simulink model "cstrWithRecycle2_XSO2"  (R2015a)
settings: Solver=ode45  StartTime=0.0  StopTime=tmax  MaxStep=0.0001  RelTol=1e-3
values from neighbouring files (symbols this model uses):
  mumax = 0.1    [cstrWithRecylce2Script.m]
  Sf = 350    [cstrWithRecylce2Script.m]
  So = 10    [cstrWithRecylce2Script.m]
  SolO2 = 9    [cstrWithRecylce2Script.m]
  SOTE = 0.20    (= 0.2)    [cstrWithRecylce2Script.m]
  Yobs = Y/(1+kd*MCRT)    [cstrWithRecylce2Script.m]
undefined symbols (not defined in the file or in its folder): amplitude, f, kd, KO2, Ks, Q, QO2, V, Xf, Xo, Y

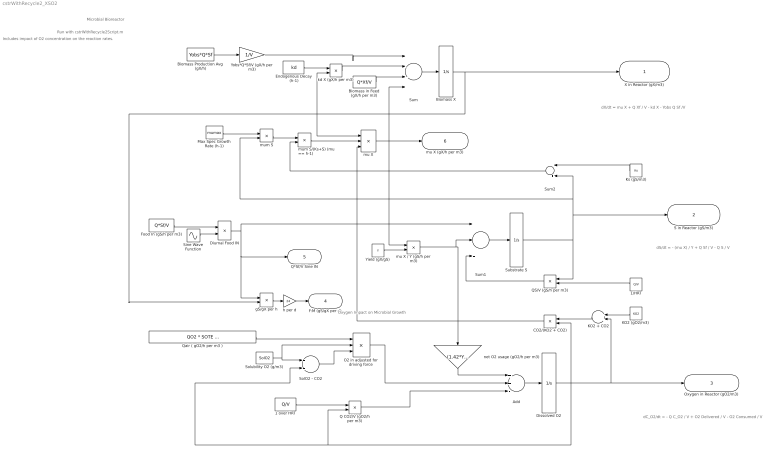
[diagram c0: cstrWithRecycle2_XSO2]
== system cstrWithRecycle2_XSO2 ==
  note: Oxygen Impact on Microbial Growth
  note: Includes impact of O2 concentration on the reaction rates.
  note: Run with cstrWithRecycle2Script.m
  note: dC_O2/dt = - Q C_O2 / V + O2 Delivered / V - O2 Consumed / V
  note: Microbial Bioreactor
  note: dS/dt = - (mu X) / Y + Q Sf / V - Q S / V
  note: dX/dt = mu X + Q Xf / V - kd X - Yobs Q Sf /V
  1 over HRT : Constant  Value=Q/V
  1/HRT : Constant  Value=Q/V
  Add : Sum  Inputs=++-
  Biomass Production Avg (gX/h) : Constant  Value=Yobs*Q*Sf
  Biomass X : Integrator  InitialCondition=Xo
  Biomass in Feed (gX/h per m3) : Constant  Value=Q*Xf/V
  CO2/(KO2 + CO2) : Product  Inputs=/*
  Dissolved O2 : Integrator  InitialCondition=9
  Diurnal Food IN : Product
  Endogenous Decay (h-1) : Constant  Value=kd
  Food In (gS/h per m3) : Constant  Value=Q*Sf/V
  "KO2 (gO2/m3) " : Constant  Value=KO2
  KO2 + CO2 : Sum
  Ks (gS/m3) : Constant  Value=Ks
  Max Spec Growth Rate (h-1) : Constant  Value=mumax
  O2 in adjusted for driving force : Product  Inputs=*/*
  Q CO2/V (gO2/h per m3) : Product
  QS/V (gS/h per m3) : Product
  Qair ( gO2/h per m3 ) : Constant  Value=QO2 * SOTE / V
  Sine Wave Function : Sin  Amplitude=amplitude  Bias=1  Frequency=0.2618  SampleTime=0
  SolO2 - CO2 : Sum  Inputs=+-
  Solubility O2 (g/m3) : Constant  Value=SolO2
  Substrate S : Integrator  InitialCondition=So
  Sum : Sum  Inputs=|--++
  Sum1 : Sum  Inputs=|+--
  Sum2 : Sum  Inputs=|++
  Yield (gX/gS) : Constant  Value=Y
  Yobs*Q*Sf/V (gX/h per m3) : Gain  Gain=1/V
  gS/gX per h : Product  Inputs=*/
  h per d : Gain  Gain=24
  kd X (gX/h per m3) : Product
  mu X : Product  Inputs=3
  mu X / Y (gS/h per m3) : Product  Inputs=*/
  mum S : Product
  mum S/(Ks+S) (mu == h-1) : Product  Inputs=*/
  net O2 usage (gO2/h per m3) : Gain  Gain=(1.42*Yobs-1/f)
  X in Reactor (gX/m3) : Outport
  S in Reactor (gS/m3) : Outport  Port=2
  Oxygen in Reactor (gO2/m3) : Outport  Port=3
  F:M (gS/gX per d) : Outport  Port=4
  Q*Sf/V Sine IN : Outport  Port=5
  mu X (gX/h per m3) : Outport  Port=6
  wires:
  Biomass X/1 -> X in Reactor (gX/m3)/1, kd X (gX/h per m3)/2, gS/gX per h/2, mu X/1
  Sum/1 -> Biomass X/1
  mu X/1 -> mu X / Y (gS/h per m3)/1, mu X (gX/h per m3)/1, Sum/4
  Max Spec Growth Rate (h-1)/1 -> mum S/1
  Sum1/1 -> Substrate S/1
  Substrate S/1 -> S in Reactor (gS/m3)/1, Sum2/2, mum S/2, QS/V (gS/h per m3)/1
  mum S/1 -> mum S/(Ks+S) (mu == h-1)/1
  Yield (gX/gS)/1 -> mu X / Y (gS/h per m3)/2
  mu X / Y (gS/h per m3)/1 -> Sum1/2, net O2 usage (gO2/h per m3)/1
  Sum2/1 -> mum S/(Ks+S) (mu == h-1)/2
  Food In (gS/h per m3)/1 -> Diurnal Food IN/1
  Sine Wave Function/1 -> Diurnal Food IN/2
  Diurnal Food IN/1 -> Sum1/1, Q*Sf/V Sine IN/1, gS/gX per h/1
  Endogenous Decay (h-1)/1 -> kd X (gX/h per m3)/1
  Ks (gS/m3)/1 -> Sum2/1
  1/HRT/1 -> QS/V (gS/h per m3)/2
  mum S/(Ks+S) (mu == h-1)/1 -> mu X/2
  Biomass Production Avg (gX/h)/1 -> Yobs*Q*Sf/V (gX/h per m3)/1
  QS/V (gS/h per m3)/1 -> Sum1/3
  Add/1 -> Dissolved O2/1
  1 over HRT/1 -> Q CO2/V (gO2/h per m3)/1
  Dissolved O2/1 -> CO2/(KO2 + CO2)/2, KO2 + CO2/2, Oxygen in Reactor (gO2/m3)/1, SolO2 - CO2/2, Q CO2/V (gO2/h per m3)/2
  "KO2 (gO2/m3) "/1 -> KO2 + CO2/1
  KO2 + CO2/1 -> CO2/(KO2 + CO2)/1
  Qair ( gO2/h per m3 )/1 -> O2 in adjusted for driving force/1
  Solubility O2 (g/m3)/1 -> O2 in adjusted for driving force/2, SolO2 - CO2/1
  h per d/1 -> F:M (gS/gX per d)/1
  gS/gX per h/1 -> h per d/1
  Biomass in Feed (gX/h per m3)/1 -> Sum/3
  kd X (gX/h per m3)/1 -> Sum/2
  CO2/(KO2 + CO2)/1 -> mu X/3
  Yobs*Q*Sf/V (gX/h per m3)/1 -> Sum/1
  net O2 usage (gO2/h per m3)/1 -> Add/1
  O2 in adjusted for driving force/1 -> Add/2
  Q CO2/V (gO2/h per m3)/1 -> Add/3
  SolO2 - CO2/1 -> O2 in adjusted for driving force/3
